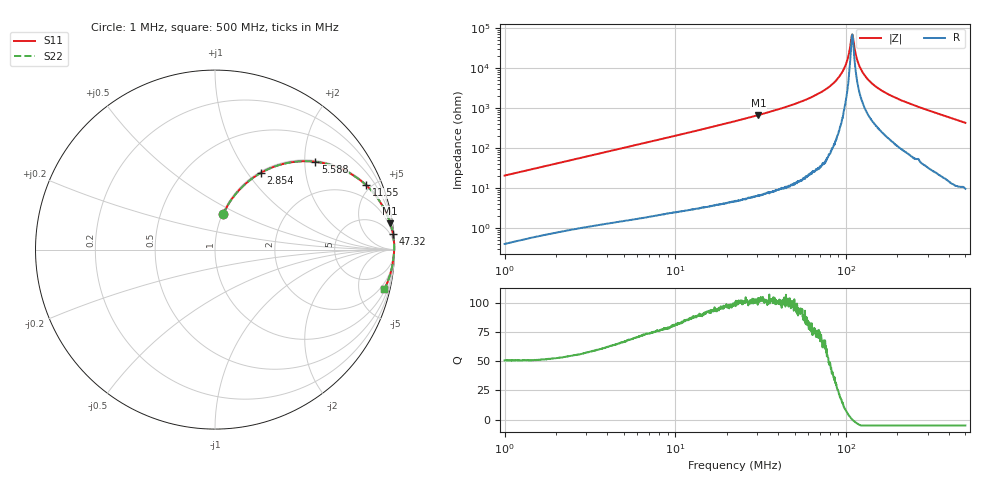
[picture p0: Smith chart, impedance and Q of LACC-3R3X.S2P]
!s-Parameter Generated by FASTRON Sdn. Bhd.
!FASTRON P/N : LACC-3R3X
!Keysight Technologies,E4991B,MY54100416,A.01.15
!Date: Wed Mar 18 09:08:44 2026
!Version  : Rev00 Wed Mar 18 09:08:44 2026
!Data & Calibration Information:
!PortZ  Port1:50+j0  Port2:50+j0
!When reading, reference impedance value at option line is always used.
!Remarks : This data is being provided solely for informational purposes.
!Freq	S11	S21	S12	S22
# Hz S dB R 50
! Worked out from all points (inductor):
!   1601 points, 1 MHz to 500 MHz, reference 50 ohm
!   read as one part in series: L = 3.26 uH near 1.032 MHz
!   highest Q = 103 at 30.63 MHz (marker M1), where L = 3.44 uH
!   self-resonance near 108.7 MHz
!   S11 on the Smith chart (normalised r, x): 1 MHz: 1.01, +0.41; 2.854 MHz: 1.02, +1.16; 5.588 MHz: 1.03, +2.26; 11.55 MHz: 1.05, +4.68; 47.32 MHz: 1, +23; 500 MHz: 1.19, -8.49
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1000000  -13.95 77.3  -0.21 -11.6  -0.21 -11.6  -13.95 77.3
2820919  -6.14 59.4  -1.30 -29.6  -1.30 -29.6  -6.14 59.4
2853982  -6.06 59.2  -1.32 -29.8  -1.32 -29.8  -6.06 59.2
5588269  -2.58 41.2  -3.63 -48.0  -3.63 -48.0  -2.58 41.2
7957584  -1.47 31.7  -5.59 -57.6  -5.59 -57.6  -1.47 31.7
1.155366e7  -0.76 23.0  -8.15 -66.3  -8.15 -66.3  -0.76 23.0
2.236068e7  -0.21 12.1  -13.58 -77.3  -13.58 -77.3  -0.21 12.1
3.062812e7  -0.11 8.6  -16.52 -80.9  -16.52 -80.9  -0.11 8.6
4.732038e7  -0.04 4.9  -21.29 -84.5  -21.29 -84.5  -0.04 4.9
6.307767e7  -0.02 3.1  -25.46 -86.2  -25.46 -86.2  -0.02 3.1
7.870937e7  -0.01 1.8  -30.20 -87.1  -30.20 -87.1  -0.01 1.8
9.158278e7  -0.01 0.9  -35.79 -86.4  -35.79 -86.4  -0.01 0.9
9.97527e7  -0.01 0.5  -41.73 -82.3  -41.73 -82.3  -0.01 0.5
1.025021e8  -0.01 0.3  -44.95 -77.8  -44.95 -77.8  -0.01 0.3
1.065617e8  -0.01 0.1  -52.63 -56.1  -52.63 -56.1  -0.01 0.1
1.086514e8  -0.01 0.0  -56.65 -4.5  -56.65 -4.5  -0.01 0.0
1.107821e8  -0.01 -0.1  -52.91 46.9  -52.91 46.9  -0.01 -0.1
1.18344e8  -0.02 -0.4  -41.97 75.5  -41.97 75.5  -0.02 -0.4
1.27408e8  -0.02 -0.8  -36.64 80.0  -36.64 80.0  -0.02 -0.8
1.453951e8  -0.03 -1.5  -31.46 82.0  -31.46 82.0  -0.03 -1.5
1.77937e8  -0.04 -2.6  -26.71 82.8  -26.71 82.8  -0.04 -2.6
5e8  -0.28 -13.2  -12.84 75.5  -12.84 75.5  -0.28 -13.2
